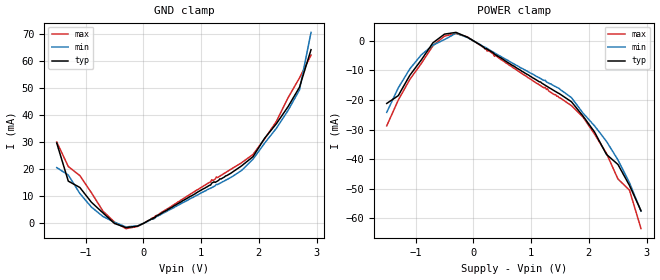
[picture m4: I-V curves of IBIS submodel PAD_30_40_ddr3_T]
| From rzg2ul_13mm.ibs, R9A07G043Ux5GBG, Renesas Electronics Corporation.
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[Submodel]  PAD_30_40_ddr3_T
Submodel_type Dynamic_clamp
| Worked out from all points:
|   GND clamp passes 1 mA (typ) near -0.10 V on its own axis
[GND Clamp]
| Voltage   I(typ)   I(min)   I(max)
-1.5V     29.69mA    20.63mA    30.08mA
-1.3V     15.63mA    17.88mA    21.03mA
-1.1V     13.29mA    11.07mA    17.68mA
-700mV    3.906mA    2.584mA    4.56mA
-500mV    -10uA      438.6uA    517.5uA
-300mV    -1.536mA   -1.286mA   -1.928mA
-100mV    -991.3uA   -903.9uA   -1.109mA
1.51V     18.47mA    16.91mA    19.93mA
1.9V      24.67mA    23.73mA    25.5mA
2.305V    36.85mA    35.17mA    37.71mA
2.705V    50.33mA    49.35mA    53.77mA
2.905V    64.2mA     70.58mA    62.19mA
[POWER Clamp]
| Voltage   I(typ)   I(min)   I(max)
-1.5V     -21.19mA   -24.2mA    -28.75mA
-1.3V     -18.54mA   -15.91mA   -20.04mA
-1.1V     -11.67mA   -9.495mA   -13.06mA
-700mV    -690.7uA   -1.484mA   -1.658mA
-300mV    2.834mA    2.556mA    2.453mA
-100mV    1.177mA    1.08mA     1.283mA
1.485V    -17.82mA   -16.12mA   -19.22mA
1.9V      -25.45mA   -24.45mA   -25.79mA
2.305V    -38.39mA   -33.97mA   -38.05mA
2.505V    -41.82mA   -40.26mA   -46.73mA
2.705V    -48.91mA   -48.01mA   -50.51mA
2.905V    -57.5mA    -57.61mA   -63.52mA
